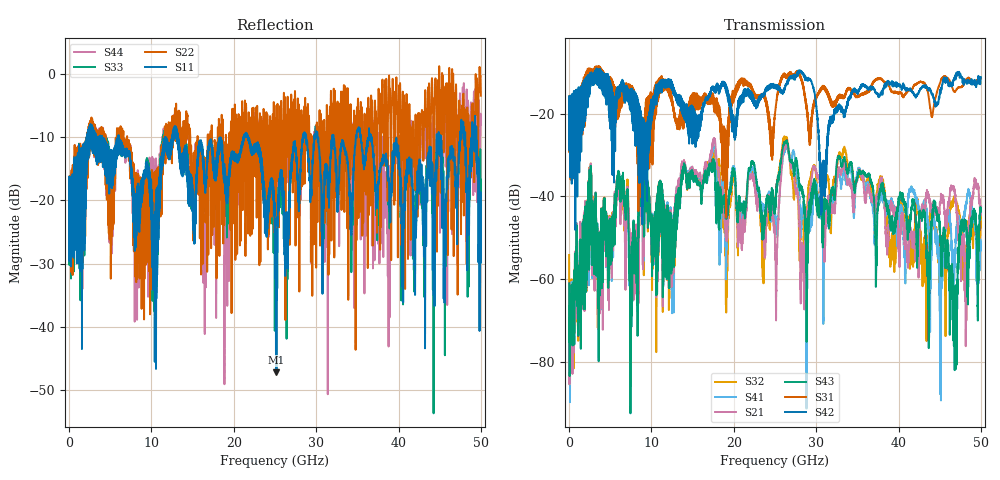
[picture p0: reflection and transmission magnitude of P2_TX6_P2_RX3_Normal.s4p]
!Keysight Technologies,N5225B,MY57041031,A.13.20.10
!Date: Friday, May 31, 2019 11:31:15
!Correction: S11(Full 4 Port(1,2,3,4))
!S12(Full 4 Port(1,2,3,4))
!S13(Full 4 Port(1,2,3,4))
!S14(Full 4 Port(1,2,3,4))
!S21(Full 4 Port(1,2,3,4))
!S22(Full 4 Port(1,2,3,4))
!S23(Full 4 Port(1,2,3,4))
!S24(Full 4 Port(1,2,3,4))
!S31(Full 4 Port(1,2,3,4))
!S32(Full 4 Port(1,2,3,4))
!S33(Full 4 Port(1,2,3,4))
!S34(Full 4 Port(1,2,3,4))
!S41(Full 4 Port(1,2,3,4))
!S42(Full 4 Port(1,2,3,4))
!S43(Full 4 Port(1,2,3,4))
!S44(Full 4 Port(1,2,3,4))
!S4P File: Measurements: <S11,S12,S13,S14>,
!<S21,S22,S23,S24>,
!<S31,S32,S33,S34>,
!<S41,S42,S43,S44>:
# Hz S  dB  R 50.0
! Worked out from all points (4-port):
!   5000 points, 10 MHz to 50 GHz, reference 50 ohm
!   strongest paths, dB at 10 MHz, 12.51 GHz, 25.01 GHz, 37.51 GHz, 50 GHz:
!     S42: -19.3, -14.1, -13.3, -15.3, -11.2
!     S31: -19.3, -16.8, -20.0, -11.6, -11.4
!     S43: -61.1, -57.7, -41.0, -43.1, -43.1
!     S21: -61.2, -60.4, -52.9, -39.8, -42.3
!     S41: -61.6, -68.3, -44.8, -42.3, -51.0
!     S32: -54.2, -55.3, -41.3, -37.4, -43.8
!   lowest |S11| = -47.2 dB at 25.18 GHz (marker M1), VSWR 1.01, Z = 50 - j0.438 ohm
!   |S11| at or under -10 dB: 13.21 GHz to 21.18 GHz (7.966 GHz wide, 46.3 % of centre); 21.74 GHz to 28.38 GHz (6.64 GHz wide, 26.5 % of centre); 36.76 GHz to 44.63 GHz (7.869 GHz wide, 19.3 % of centre)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
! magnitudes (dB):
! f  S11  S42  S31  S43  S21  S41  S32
! 10 MHz  -19.4  -19.3  -19.3  -61.1  -61.2  -61.6  -54.2
! 2.59 GHz  -9.8  -13.4  -12.4  -33.9  -33.0  -33.6  -33.2
! 25.18 GHz  -47.2  -13.8  -16.9  -39.1  -62.8  -48.2  -38.8
! 26.34 GHz  -25.2  -13.0  -11.0  -26.6  -27.6  -28.3  -25.6
! 28.33 GHz  -10.4  -10.0  -12.7  -38.4  -54.7  -42.8  -43.1
! 46.8 GHz  -13.6  -11.5  -14.6  -61.8  -38.5  -53.5  -40.2
! 50 GHz  -22.9  -11.2  -11.4  -43.1  -42.3  -51.0  -43.8
